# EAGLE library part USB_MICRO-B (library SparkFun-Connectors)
USB Type Micro-B Connector Male/female and PTH/SMT variants SparkFun Products: SparkFun microB USB Breakout SparkFun USB microB Plug Breakout SparkFun ESP8266 Thing
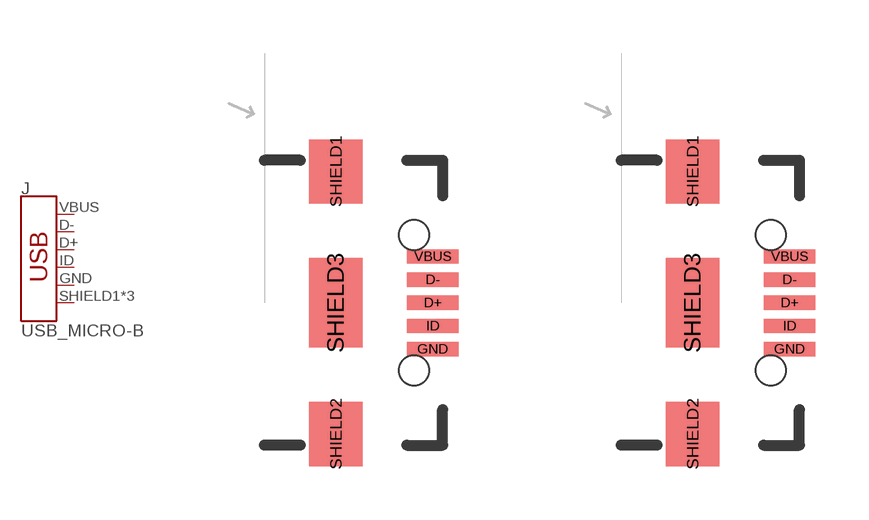
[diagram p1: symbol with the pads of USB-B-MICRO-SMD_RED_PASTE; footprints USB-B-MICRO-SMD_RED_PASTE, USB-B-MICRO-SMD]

Designator prefix J

## USB_MICRO-BREDUCED_PASTE (PROD_ID: CONN-11752)  [USB-B-MICRO-SMD_RED_PASTE]
D+  D+
D-  D-
GND  GND  pwr
ID  ID
SHIELD1  SHIELD
SHIELD2  SHIELD
SHIELD3  SHIELD
VBUS  VBUS  pwr

## USB_MICRO-B_FEMALE-SMT (PROD_ID: CONN-11752)  [USB-B-MICRO-SMD]
Pads as for USB-B-MICRO-SMD_RED_PASTE

## USB_MICRO-B_FEMALE-SMT-VERT (PROD_ID: CONN-13534; VALUE: WM9734TR-ND)  [USB-B-MICRO-SMD_VERT]
D+  D+
D-  D-
GND  GND  pwr
ID  ID
P1  SHIELD
P2  SHIELD
P3  SHIELD
VBUS  VBUS  pwr

## USB_MICRO-B_HALF_PTH_MILL (PROD_ID: CONN-13711)  [USB-MICROB-PTH-MILL]
D+  D+
D-  D-
GND  GND  pwr
ID  ID
SHIELD  SHIELD
SHIELD2  SHIELD
SHIELD3  SHIELD
SHIELD4  SHIELD
SHIELD5  SHIELD
SHIELD6  SHIELD
SHIELD7  SHIELD
SHIELD8  SHIELD
SHIELD9  SHIELD
SHIELD10  SHIELD
VBUS  VBUS  pwr

## USB_MICRO-B_MALE-VERT (PROD_ID: CONN-09900)  [USB_MICROB_VERTICAL]
D+  D+
D-  D-
GND  GND  pwr
ID  ID
SHLD1  SHIELD
SHLD2  SHIELD
SHLD3  SHIELD
SHLD4  SHIELD
VBUS  VBUS  pwr

## USB_MICRO-B_SMT (PROD_ID: CONN-09505; SF_ID: PRT-08533)  [USB-MICROB]
D+  D+
D-  D-
GND  GND  pwr
ID  ID
MT1  SHIELD
MT2  SHIELD
P$1  SHIELD
P$2  SHIELD
VBUS  VBUS  pwr

## Footprint USB-B-MICRO-SMD_RED_PASTE (pad centres in mm)
USB - microB SMD Reduced Paste 70% paste area under D+ D- USBID pins for applications where those pins aren't required, to reduce the likelihood of bridges. Specifications: Pin count:5 Datasheet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
smd 1.45 x 0.4: D+ 2.725,0; D- 2.725,0.65; GND 2.725,-1.3; ID 2.725,-0.65; VBUS 2.725,1.3
smd 1.5 x 1.8: SHIELD1 0,3.685; SHIELD2 0,-3.685
smd 1.5 x 2.5: SHIELD3 0,0
hole 0.85 at 2.2,1.9
hole 0.85 at 2.2,-1.9

## Footprint USB-B-MICRO-SMD (pad centres in mm)
USB - microB SMD Specifications: Pin count:5 Datasheet referenced for footprint Example device(s): USB_MICRO-B
smd 1.45 x 0.4: D+ 2.725,0; D- 2.725,0.65; GND 2.725,-1.3; ID 2.725,-0.65; VBUS 2.725,1.3
smd 1.5 x 1.8: SHIELD1 0,3.685; SHIELD2 0,-3.685
smd 1.5 x 2.5: SHIELD3 0,0
hole 0.85 at 2.2,1.9
hole 0.85 at 2.2,-1.9

## Footprint USB-B-MICRO-SMD_VERT (pad centres in mm)
smd 0.45 x 1.5: D+ 0,0; D- -0.65,0; GND 1.3,0; ID 0.65,0; VBUS -1.3,0
drill 1.016: P1 -2.8,0.25; P2 2.8,0.25
drill 1.27: P3 0,-1.9

## Footprint USB-MICROB-PTH-MILL (pad centres in mm)
smd 0.4 x 1.75: D+ 0,0; D- -0.65,0; GND 1.3,0; ID 0.65,0; VBUS -1.3,0
smd 2 x 1.46: SHIELD -2.9,0.275; SHIELD2 2.9,0.275
smd 1.425 x 2.5: SHIELD3 -0.963,-2.675; SHIELD4 0.963,-2.675
smd 1.4 x 2.1 bottom: SHIELD5 -2.731,-2.531; SHIELD7 2.729,-2.531
smd 1 x 1: SHIELD6 2.7,-2.575
smd 1.1 x 1.5: SHIELD8 -2.731,-2.731
smd 1 x 1.3 bottom: SHIELD9 -2.43,0.195; SHIELD10 2.43,0.195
